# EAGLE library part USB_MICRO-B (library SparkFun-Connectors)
USB Type Micro-B Connector Male/female and PTH/SMT variants SparkFun Products: SparkFun microB USB Breakout SparkFun USB microB Plug Breakout SparkFun ESP8266 Thing
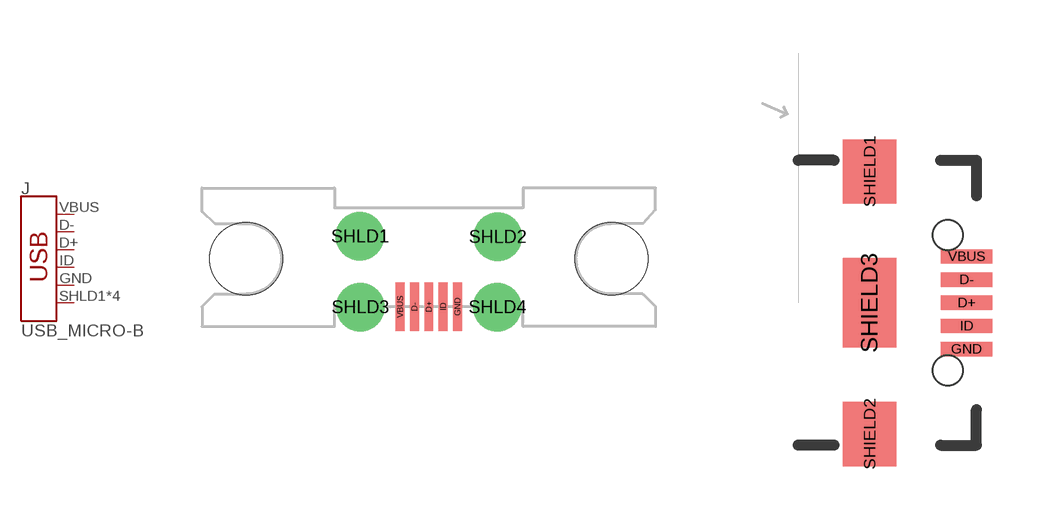
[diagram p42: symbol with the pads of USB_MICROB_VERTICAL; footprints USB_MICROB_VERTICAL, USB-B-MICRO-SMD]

Designator prefix J

## USB_MICRO-B_MALE-VERT (PROD_ID: CONN-09900)  [USB_MICROB_VERTICAL]
D+  D+
D-  D-
GND  GND  pwr
ID  ID
SHLD1  SHIELD
SHLD2  SHIELD
SHLD3  SHIELD
SHLD4  SHIELD
VBUS  VBUS  pwr

## USB_MICRO-B_FEMALE-SMT (PROD_ID: CONN-11752)  [USB-B-MICRO-SMD]
D+  D+
D-  D-
GND  GND  pwr
ID  ID
SHIELD1  SHIELD
SHIELD2  SHIELD
SHIELD3  SHIELD
VBUS  VBUS  pwr

## USB_MICRO-B_SMT (PROD_ID: CONN-09505; SF_ID: PRT-08533)  [USB-MICROB]
D+  D+
D-  D-
GND  GND  pwr
ID  ID
MT1  SHIELD
MT2  SHIELD
P$1  SHIELD
P$2  SHIELD
VBUS  VBUS  pwr

## USB_MICRO-BREDUCED_PASTE (PROD_ID: CONN-11752)  [USB-B-MICRO-SMD_RED_PASTE]
Pads as for USB-B-MICRO-SMD

## USB_MICRO-B_FEMALE-SMT-VERT (PROD_ID: CONN-13534; VALUE: WM9734TR-ND)  [USB-B-MICRO-SMD_VERT]
D+  D+
D-  D-
GND  GND  pwr
ID  ID
P1  SHIELD
P2  SHIELD
P3  SHIELD
VBUS  VBUS  pwr

## USB_MICRO-B_HALF_PTH_MILL (PROD_ID: CONN-13711)  [USB-MICROB-PTH-MILL]
D+  D+
D-  D-
GND  GND  pwr
ID  ID
SHIELD  SHIELD
SHIELD2  SHIELD
SHIELD3  SHIELD
SHIELD4  SHIELD
SHIELD5  SHIELD
SHIELD6  SHIELD
SHIELD7  SHIELD
SHIELD8  SHIELD
SHIELD9  SHIELD
SHIELD10  SHIELD
VBUS  VBUS  pwr

## Footprint USB_MICROB_VERTICAL (pad centres in mm)
USB Micro-B Plug Connector Manufacturer part #: ZX80-B-5SA Manufacturer: Hirose Specifications: Pin count: 5 main, 4 shield Datasheet referenced for footprint Example device(s): USB_Micro-B
smd 0.4 x 2.2: D+ 0,0; D- -0.65,0; GND 1.3,0; ID 0.65,0; VBUS -1.3,0
drill 1.016 pad 2.2: SHLD1 -3.121,3.183; SHLD2 3.122,3.16; SHLD3 -3.098,-0.027; SHLD4 3.108,-0.026
hole 3.3 at -8.275,2.17
hole 3.3 at 8.275,2.17

## Footprint USB-B-MICRO-SMD (pad centres in mm)
USB - microB SMD Specifications: Pin count:5 Datasheet referenced for footprint Example device(s): USB_MICRO-B
smd 1.45 x 0.4: D+ 2.725,0; D- 2.725,0.65; GND 2.725,-1.3; ID 2.725,-0.65; VBUS 2.725,1.3
smd 1.5 x 1.8: SHIELD1 0,3.685; SHIELD2 0,-3.685
smd 1.5 x 2.5: SHIELD3 0,0
hole 0.85 at 2.2,1.9
hole 0.85 at 2.2,-1.9

## Footprint USB-MICROB (pad centres in mm)
USB Type microUSB Connector-No Bossed Pins Specifications: Pin count:5 pins, 4 shield connections Example device(s): USB_Micro-B
smd 1.4 x 0.35: D+ -2.65,0; D- -2.65,-0.65; GND -2.65,1.3; ID -2.65,0.65; VBUS -2.65,-1.3
smd 1.9 x 1.8: MT1 0,-4; MT2 0,4
smd 1.9 x 1.9: P$1 0,-1.27; P$2 0,1.27

## Footprint USB-B-MICRO-SMD_RED_PASTE (pad centres in mm)
USB - microB SMD Reduced Paste 70% paste area under D+ D- USBID pins for applications where those pins aren't required, to reduce the likelihood of bridges. Specifications: Pin count:5 Datasheet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
smd 1.45 x 0.4: D+ 2.725,0; D- 2.725,0.65; GND 2.725,-1.3; ID 2.725,-0.65; VBUS 2.725,1.3
smd 1.5 x 1.8: SHIELD1 0,3.685; SHIELD2 0,-3.685
smd 1.5 x 2.5: SHIELD3 0,0
hole 0.85 at 2.2,1.9
hole 0.85 at 2.2,-1.9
